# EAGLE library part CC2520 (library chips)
2.4 GHZ IEEE 802.15.4/ZIGBEE® RF TRANSCEIVER
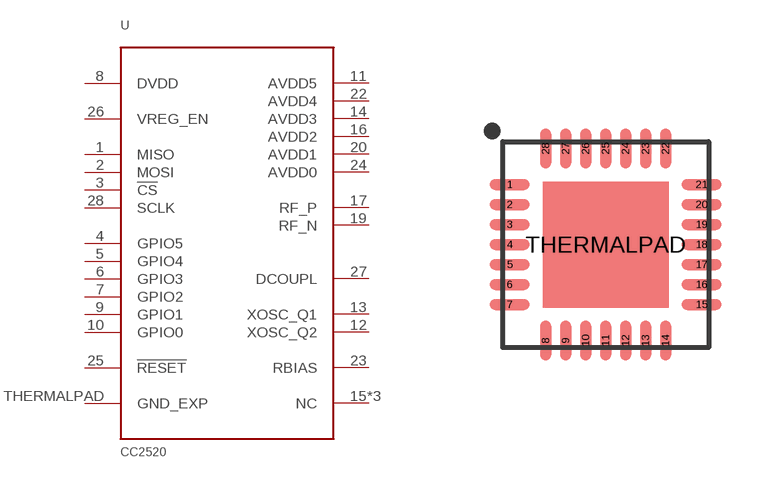
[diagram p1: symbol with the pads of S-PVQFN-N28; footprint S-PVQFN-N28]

Designator prefix U

## CC2520 (DIGIKEY: 296-22996-1-ND)  [S-PVQFN-N28]
1  MISO
2  MOSI
3  !CS
4  GPIO5
5  GPIO4
6  GPIO3
7  GPIO2
8  DVDD
9  GPIO1
10  GPIO0
11  AVDD5
12  XOSC_Q2
13  XOSC_Q1
14  AVDD3
15  NC
16  AVDD2
17  RF_P
18  NC
19  RF_N
20  AVDD1
21  NC
22  AVDD4
23  RBIAS
24  AVDD0
25  !RESET
26  VREG_EN
27  DCOUPL
28  SCLK
THERMALPAD  GND_EXP

## Footprint S-PVQFN-N28 (pad centres in mm)
5 x 5 mm QFN28 (RHD)
smd 1 x 0.28: 1 -2.4,1.5; 2 -2.4,1; 3 -2.4,0.5; 4 -2.4,0; 5 -2.4,-0.5; 6 -2.4,-1; 7 -2.4,-1.5; 15 2.4,-1.5; 16 2.4,-1; 17 2.4,-0.5; 18 2.4,0; 19 2.4,0.5; 20 2.4,1; 21 2.4,1.5
smd 0.28 x 1: 8 -1.5,-2.4; 9 -1,-2.4; 10 -0.5,-2.4; 11 0,-2.4; 12 0.5,-2.4; 13 1,-2.4; 14 1.5,-2.4; 22 1.5,2.4; 23 1,2.4; 24 0.5,2.4; 25 0,2.4; 26 -0.5,2.4; 27 -1,2.4; 28 -1.5,2.4
smd 3.15 x 3.15: THERMALPAD 0,0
